| IBIS File LibisMaker.ibs
| Cadence Design Systems, Inc. 2024
[IBIS Ver]   7.0
[File name]   ln2-mh.ibs
[File rev]   1.7.1
[Date]   Wed Aug 12 20:25:11 PDT 2026
[Source]   Lattice Semiconductor Process
[Notes]   Device: LN2-MH-16
   CBG484   Final
   Device: LN2-MH-20
   CBG484   Final
   Lattice Semiconductor has worked hard to ensure the
   models below are accurate and complete.  However, the
   data below was generated using simulation of the
   input/output model files for the silicon.  Therefore,
   the data below is for reference and initial design
   purposes only.
   Lattice Semiconductor grants permission to use this
   data for use in printed circuit design using this
   Lattice programmable logic device.  Other use of this
   code, including the selling or duplication of any
   portion is strictly prohibited.
|   NAMING CONVENTION
   The IBIS [Model] header is limited by the specification to a
   total of characters.  With such a set of characters available
   for naming models it becomes important to attempt to
   meaningfully encode the IO standards so they fit within the
   twenty character limit.  It would seem that twenty characters
   would provide room enough for describing IO's.  However, the
   PLD IO structure continues to grow more and more complex.  The
   complexity is making the twenty characters insuffiently
   descriptive.  In order to overcome this issue the naming
   convention described below is implemented to resolve the issue.
The twenty character space is managed as follows:
   bbbvvvsdddprttmkoixx
   b = standard
   v = voltage (x.xx V)
   s = slew code
   d = drive (xx.x ma)
   p = pullmode code
   r = impedance
   t = termination code
   m = mipi hard dphy mode
   k = bank code
   o = diff resistor code
   i = diff  current code
   x = reserved
   standard
   lvcmos   lvc
   sstl135   ss1
   sstl135d   s1d
   hsul12   hs1
   hsul12d   h1d
   lvds   lvs
   lvdse   lve
   slvs   svs
   sublvds   slv
   sublvdse   sle
   mipi_dphy   mip
   pod   pod
   podd   pdd
   lvstl_i   ls1
   lvstl_ii   ls2
   lvstld_i   l1d
   lvstld_ii   l2d
   vref_driver   vr1
   slew
   na   a
   fast   f
   slow   s
   drive
   2   020
   4   040
   6   060
   8   080
   12   120
   50rs   r50
   34_ohm   034
   40_ohm   040
   48_ohm   048
   60_ohm   060
   80_ohm   080
   120_ohm   120
   240_ohm   240
   na   xxx
   pullmode
   none   a
   failsafe   a
   up   b
   down   c
   keeper   d
   i3c   i
   impedance
   off   a
   termination
   off   aa
   34   bb
   40   cc
   48   dd
   60   ee
   80   ff
   120   gg
   240   hh
   mipi hard dphy mode
   off   a
   lp   l
   hs   h
   bank
   wrio   a
   hpio   h
   differential resistor
   off   a
   100   b
   differential current
   NA   a
   2.0   b
   3.5   c
   Reserved   IO type
   in   input only
   ou   output
   io   I/O
   od   Open drain
   ic   Inverting differential input
   (signal name only)
   it   Non-Inverting differential
   input (signal name only)
   on   Inverting differential output
   (signal name only)
   op   Non-Inverting differential output
   (signal name only)
   bn   Inverting differential I/O
   (signal name only)
   bp   Non-Inverting differential I/O
   (signal name only)
   All the IO models are generated with pull mode set to none.
   Lattice Semiconductor Corporation
   5555 NE Moore Court
   Hillsboro, OR 97214
   U.S.A
   TEL: 1-800-Lattice (USA and Canada)
   408-826-6000 (other locations)
   All the IO models are generated with pull mode set to none.
   Lattice Semiconductor Corporation
   5555 NE Moore Court
   Hillsboro, OR 97214
   U.S.A
   TEL: 1-800-Lattice (USA and Canada)
   408-826-6000 (other locations)
   web: http://www.latticesemi.com/
   email: techsupport@latticesemi.com
[Disclaimer] This IBIS source code is intended as a design reference
   which illustrates how the Lattice Semiconductor device operates.
   It is the user's responsibility to verify their design for
   consistency and functionality through the use of formal
   verification methods.  Lattice Semiconductor provides no warranty
   regarding the use or functionality of this data.
[Copyright]  Copyright 2025 by Lattice Semiconductor Corporation
|   Component LN2-MH
[Component] LN2-MH
[Manufacturer] Lattice Semiconductor Corp.
[Package]
|CBG484_20ES1
| variable   typ   min   max
R_pkg   0.05332   0.013842   0.098293
L_pkg   2.82e-9   3.896e-10   5.244e-9
C_pkg   1.436e-12   6.976e-13   2.382e-12
|CBG484_16
| variable   typ   min   max
|R_pkg   0.3858   0.054089   0.93239
|L_pkg   2.783e-9   4.558e-10   6.119e-9
|C_pkg   1.392e-12   3.932e-13   2.869e-12
|CBG484_20
| variable   typ   min   max
|R_pkg   0.3858   0.054089   0.93239
|L_pkg   2.783e-9   4.558e-10   6.119e-9
|C_pkg   1.392e-12   3.932e-13   2.869e-12
[Pin]  signal_name   model_name   R_pin   L_pin   C_pin
1   lvc180axxxaaaaaaaain   lvc180axxxaaaaaaaain
2   lvc180axxxbaaaaaaain   lvc180axxxbaaaaaaain
3   lvc180axxxcaaaaaaain   lvc180axxxcaaaaaaain
4   lvc180axxxdaaaaaaain   lvc180axxxdaaaaaaain
5   lvc250axxxaaaaaaaain   lvc250axxxaaaaaaaain
6   lvc250axxxbaaaaaaain   lvc250axxxbaaaaaaain
7   lvc250axxxcaaaaaaain   lvc250axxxcaaaaaaain
8   lvc250axxxdaaaaaaain   lvc250axxxdaaaaaaain
9   lvc330axxxaaaaaaaain   lvc330axxxaaaaaaaain
10   lvc330axxxbaaaaaaain   lvc330axxxbaaaaaaain
11   lvc330axxxcaaaaaaain   lvc330axxxcaaaaaaain
12   lvc330axxxdaaaaaaain   lvc330axxxdaaaaaaain
13   lvc120axxxaaaaaaaain   lvc120axxxaaaaaaaain
14   lvc120axxxbaaaaaaain   lvc120axxxbaaaaaaain
15   lvc120axxxcaaaaaaain   lvc120axxxcaaaaaaain
16   lvc120axxxdaaaaaaain   lvc120axxxdaaaaaaain
17   lvc120axxxaaaaahaain   lvc120axxxaaaaahaain
18   lvc120axxxbaaaahaain   lvc120axxxbaaaahaain
19   lvc120axxxcaaaahaain   lvc120axxxcaaaahaain
20   lvc120axxxdaaaahaain   lvc120axxxdaaaahaain
21   lvc120axxxiaaaahaain   lvc120axxxiaaaahaain
22   lvc180axxxaaaaahaain   lvc180axxxaaaaahaain
23   lvc180axxxbaaaahaain   lvc180axxxbaaaahaain
24   lvc180axxxcaaaahaain   lvc180axxxcaaaahaain
25   lvc180axxxdaaaahaain   lvc180axxxdaaaahaain
26   lvc180axxxiaaaahaain   lvc180axxxiaaaahaain
27   lvc090axxxaaaaahaain   lvc090axxxaaaaahaain
28   lvc090axxxbaaaahaain   lvc090axxxbaaaahaain
29   lvc090axxxcaaaahaain   lvc090axxxcaaaahaain
30   lvc090axxxdaaaahaain   lvc090axxxdaaaahaain
31   lvc100axxxaaaaahaain   lvc100axxxaaaaahaain
32   lvc100axxxbaaaahaain   lvc100axxxbaaaahaain
33   lvc100axxxcaaaahaain   lvc100axxxcaaaahaain
34   lvc100axxxdaaaahaain   lvc100axxxdaaaahaain
35   ls1110axxxaabbahaain   ls1110axxxaabbahaain
36   ls1110axxxaaccahaain   ls1110axxxaaccahaain
37   ls1110axxxaaddahaain   ls1110axxxaaddahaain
38   ls1110axxxaaeeahaain   ls1110axxxaaeeahaain
39   ls1110axxxaaffahaain   ls1110axxxaaffahaain
40   ls1110axxxaaggahaain   ls1110axxxaaggahaain
41   ls1110axxxaahhahaain   ls1110axxxaahhahaain
42   ls2110axxxaabbahaain   ls2110axxxaabbahaain
43   ls2110axxxaaccahaain   ls2110axxxaaccahaain
44   ls2110axxxaaddahaain   ls2110axxxaaddahaain
45   ls2110axxxaaeeahaain   ls2110axxxaaeeahaain
46   ls2110axxxaaffahaain   ls2110axxxaaffahaain
47   ls2110axxxaaggahaain   ls2110axxxaaggahaain
48   ls2110axxxaahhahaain   ls2110axxxaahhahaain
49   hs1120axxxaaaaahaain   hs1120axxxaaaaahaain
50   hs1120axxxaaccahaain   hs1120axxxaaccahaain
51   hs1120axxxaaeeahaain   hs1120axxxaaeeahaain
52   pod110axxxaabbahaain   pod110axxxaabbahaain
53   pod110axxxaaccahaain   pod110axxxaaccahaain
54   pod110axxxaaddahaain   pod110axxxaaddahaain
55   pod110axxxaaeeahaain   pod110axxxaaeeahaain
56   pod110axxxaaffahaain   pod110axxxaaffahaain
57   pod110axxxaaggahaain   pod110axxxaaggahaain
58   pod110axxxaahhahaain   pod110axxxaahhahaain
59   pod120axxxaabbahaain   pod120axxxaabbahaain
60   pod120axxxaaccahaain   pod120axxxaaccahaain
61   pod120axxxaaddahaain   pod120axxxaaddahaain
62   pod120axxxaaeeahaain   pod120axxxaaeeahaain
63   pod120axxxaaffahaain   pod120axxxaaffahaain
64   pod120axxxaaggahaain   pod120axxxaaggahaain
65   pod120axxxaahhahaain   pod120axxxaahhahaain
66   ss1135axxxaaaaahaain   ss1135axxxaaaaahaain
67   ss1135axxxaaccahaain   ss1135axxxaaccahaain
68   ss1135axxxaaeeahaain   ss1135axxxaaeeahaain
69   l1d110axxxaabbahaait   l1d110axxxaabbahaain
70   l1d110axxxaabbahaaic   l1d110axxxaabbahaain
71   l1d110axxxaaccahaait   l1d110axxxaaccahaain
72   l1d110axxxaaccahaaic   l1d110axxxaaccahaain
73   l1d110axxxaaddahaait   l1d110axxxaaddahaain
74   l1d110axxxaaddahaaic   l1d110axxxaaddahaain
75   l1d110axxxaaeeahaait   l1d110axxxaaeeahaain
76   l1d110axxxaaeeahaaic   l1d110axxxaaeeahaain
77   l1d110axxxaaffahaait   l1d110axxxaaffahaain
78   l1d110axxxaaffahaaic   l1d110axxxaaffahaain
79   l1d110axxxaaggahaait   l1d110axxxaaggahaain
80   l1d110axxxaaggahaaic   l1d110axxxaaggahaain
81   l1d110axxxaahhahaait   l1d110axxxaahhahaain
82   l1d110axxxaahhahaaic   l1d110axxxaahhahaain
83   l2d110axxxaabbahaait   l2d110axxxaabbahaain
84   l2d110axxxaabbahaaic   l2d110axxxaabbahaain
85   l2d110axxxaaccahaait   l2d110axxxaaccahaain
86   l2d110axxxaaccahaaic   l2d110axxxaaccahaain
87   l2d110axxxaaddahaait   l2d110axxxaaddahaain
88   l2d110axxxaaddahaaic   l2d110axxxaaddahaain
89   l2d110axxxaaeeahaait   l2d110axxxaaeeahaain
90   l2d110axxxaaeeahaaic   l2d110axxxaaeeahaain
91   l2d110axxxaaffahaait   l2d110axxxaaffahaain
92   l2d110axxxaaffahaaic   l2d110axxxaaffahaain
93   l2d110axxxaaggahaait   l2d110axxxaaggahaain
94   l2d110axxxaaggahaaic   l2d110axxxaaggahaain
95   l2d110axxxaahhahaait   l2d110axxxaahhahaain
96   l2d110axxxaahhahaaic   l2d110axxxaahhahaain
97   h1d120axxxaaaaahaait   h1d120axxxaaaaahaain
98   h1d120axxxaaaaahaaic   h1d120axxxaaaaahaain
99   h1d120axxxaaaaahbait   h1d120axxxaaaaahbain
100   h1d120axxxaaaaahbaic   h1d120axxxaaaaahbain
101   h1d120axxxaaccahaait   h1d120axxxaaccahaain
102   h1d120axxxaaccahaaic   h1d120axxxaaccahaain
103   h1d120axxxaaccahbait   h1d120axxxaaccahbain
104   h1d120axxxaaccahbaic   h1d120axxxaaccahbain
105   h1d120axxxaaeeahaait   h1d120axxxaaeeahaain
106   h1d120axxxaaeeahaaic   h1d120axxxaaeeahaain
107   h1d120axxxaaeeahbait   h1d120axxxaaeeahbain
108   h1d120axxxaaeeahbaic   h1d120axxxaaeeahbain
109   pdd110axxxaabbahaait   pdd110axxxaabbahaain
110   pdd110axxxaabbahaaic   pdd110axxxaabbahaain
111   pdd110axxxaaccahaait   pdd110axxxaaccahaain
112   pdd110axxxaaccahaaic   pdd110axxxaaccahaain
113   pdd110axxxaaddahaait   pdd110axxxaaddahaain
114   pdd110axxxaaddahaaic   pdd110axxxaaddahaain
115   pdd110axxxaaeeahaait   pdd110axxxaaeeahaain
116   pdd110axxxaaeeahaaic   pdd110axxxaaeeahaain
117   pdd110axxxaaffahaait   pdd110axxxaaffahaain
118   pdd110axxxaaffahaaic   pdd110axxxaaffahaain
119   pdd110axxxaaggahaait   pdd110axxxaaggahaain
120   pdd110axxxaaggahaaic   pdd110axxxaaggahaain
121   pdd110axxxaahhahaait   pdd110axxxaahhahaain
122   pdd110axxxaahhahaaic   pdd110axxxaahhahaain
123   pdd120axxxaabbahaait   pdd120axxxaabbahaain
124   pdd120axxxaabbahaaic   pdd120axxxaabbahaain
125   pdd120axxxaaccahaait   pdd120axxxaaccahaain
126   pdd120axxxaaccahaaic   pdd120axxxaaccahaain
127   pdd120axxxaaddahaait   pdd120axxxaaddahaain
128   pdd120axxxaaddahaaic   pdd120axxxaaddahaain
129   pdd120axxxaaeeahaait   pdd120axxxaaeeahaain
130   pdd120axxxaaeeahaaic   pdd120axxxaaeeahaain
131   pdd120axxxaaffahaait   pdd120axxxaaffahaain
132   pdd120axxxaaffahaaic   pdd120axxxaaffahaain
133   pdd120axxxaaggahaait   pdd120axxxaaggahaain
134   pdd120axxxaaggahaaic   pdd120axxxaaggahaain
135   pdd120axxxaahhahaait   pdd120axxxaahhahaain
136   pdd120axxxaahhahaaic   pdd120axxxaahhahaain
137   s1d135axxxaaaaahaait   s1d135axxxaaaaahaain
138   s1d135axxxaaaaahaaic   s1d135axxxaaaaahaain
139   s1d135axxxaaaaahbait   s1d135axxxaaaaahbain
140   s1d135axxxaaaaahbaic   s1d135axxxaaaaahbain
141   s1d135axxxaaccahaait   s1d135axxxaaccahaain
142   s1d135axxxaaccahaaic   s1d135axxxaaccahaain
143   s1d135axxxaaccahbait   s1d135axxxaaccahbain
144   s1d135axxxaaccahbaic   s1d135axxxaaccahbain
145   s1d135axxxaaeeahaait   s1d135axxxaaeeahaain
146   s1d135axxxaaeeahaaic   s1d135axxxaaeeahaain
147   s1d135axxxaaeeahbait   s1d135axxxaaeeahbain
148   s1d135axxxaaeeahbaic   s1d135axxxaaeeahbain
149   slv180axxxaaaaahaait   slv180axxxaaaaahaain
150   slv180axxxaaaaahaaic   slv180axxxaaaaahaain
151   slv180axxxaaaaahbait   slv180axxxaaaaahbain
152   slv180axxxaaaaahbaic   slv180axxxaaaaahbain
153   svs120axxxaaaaahaait   svs120axxxaaaaahaain
154   svs120axxxaaaaahaaic   svs120axxxaaaaahaain
155   svs120axxxaaaaahbait   svs120axxxaaaaahbain
156   svs120axxxaaaaahbaic   svs120axxxaaaaahbain
157   mip120axxxaaaaahbait   mip120axxxaaaaahbain
158   mip120axxxaaaaahbaic   mip120axxxaaaaahbain
159   lvs180axxxaaaaahaait   lvs180axxxaaaaahaain
160   lvs180axxxaaaaahaaic   lvs180axxxaaaaahaain
161   lvs180axxxaaaaahbait   lvs180axxxaaaaahbain
162   lvs180axxxaaaaahbaic   lvs180axxxaaaaahbain
163   lvc120f040aaaaahaaou   lvc120f040aaaaahaaou
164   lvc120f080aaaaahaaou   lvc120f080aaaaahaaou
165   lvc120f120aaaaahaaou   lvc120f120aaaaahaaou
166   lvc120s040aaaaahaaou   lvc120s040aaaaahaaou
167   lvc120s080aaaaahaaou   lvc120s080aaaaahaaou
168   lvc120s120aaaaahaaou   lvc120s120aaaaahaaou
169   lvc180f040aaaaahaaou   lvc180f040aaaaahaaou
170   lvc180f080aaaaahaaou   lvc180f080aaaaahaaou
171   lvc180f120aaaaahaaou   lvc180f120aaaaahaaou
172   lvc180fr50aaaaahaaou   lvc180fr50aaaaahaaou
173   lvc180s040aaaaahaaou   lvc180s040aaaaahaaou
174   lvc180s080aaaaahaaou   lvc180s080aaaaahaaou
175   lvc180s120aaaaahaaou   lvc180s120aaaaahaaou
176   lvc180sr50aaaaahaaou   lvc180sr50aaaaahaaou
177   lvc090f020aaaaahaaou   lvc090f020aaaaahaaou
178   lvc090f040aaaaahaaou   lvc090f040aaaaahaaou
179   lvc090f080aaaaahaaou   lvc090f080aaaaahaaou
180   lvc090s020aaaaahaaou   lvc090s020aaaaahaaou
181   lvc090s040aaaaahaaou   lvc090s040aaaaahaaou
182   lvc090s080aaaaahaaou   lvc090s080aaaaahaaou
183   lvc100f020aaaaahaaou   lvc100f020aaaaahaaou
184   lvc100f040aaaaahaaou   lvc100f040aaaaahaaou
185   lvc100f080aaaaahaaou   lvc100f080aaaaahaaou
186   lvc100s020aaaaahaaou   lvc100s020aaaaahaaou
187   lvc100s040aaaaahaaou   lvc100s040aaaaahaaou
188   lvc100s080aaaaahaaou   lvc100s080aaaaahaaou
189   lvc180f040aaaaaaaaou   lvc180f040aaaaaaaaou
190   lvc180f080aaaaaaaaou   lvc180f080aaaaaaaaou
191   lvc180f120aaaaaaaaou   lvc180f120aaaaaaaaou
192   lvc180fr50aaaaaaaaou   lvc180fr50aaaaaaaaou
193   lvc180s040aaaaaaaaou   lvc180s040aaaaaaaaou
194   lvc180s080aaaaaaaaou   lvc180s080aaaaaaaaou
195   lvc180s120aaaaaaaaou   lvc180s120aaaaaaaaou
196   lvc180sr50aaaaaaaaou   lvc180sr50aaaaaaaaou
197   lvc250f040aaaaaaaaou   lvc250f040aaaaaaaaou
198   lvc250f080aaaaaaaaou   lvc250f080aaaaaaaaou
199   lvc250f120aaaaaaaaou   lvc250f120aaaaaaaaou
200   lvc250fr50aaaaaaaaou   lvc250fr50aaaaaaaaou
201   lvc250s040aaaaaaaaou   lvc250s040aaaaaaaaou
202   lvc250s080aaaaaaaaou   lvc250s080aaaaaaaaou
203   lvc250s120aaaaaaaaou   lvc250s120aaaaaaaaou
204   lvc250sr50aaaaaaaaou   lvc250sr50aaaaaaaaou
205   lvc330f040aaaaaaaaou   lvc330f040aaaaaaaaou
206   lvc330f080aaaaaaaaou   lvc330f080aaaaaaaaou
207   lvc330f120aaaaaaaaou   lvc330f120aaaaaaaaou
208   lvc330fr50aaaaaaaaou   lvc330fr50aaaaaaaaou
209   lvc330s040aaaaaaaaou   lvc330s040aaaaaaaaou
210   lvc330s080aaaaaaaaou   lvc330s080aaaaaaaaou
211   lvc330s120aaaaaaaaou   lvc330s120aaaaaaaaou
212   lvc330sr50aaaaaaaaou   lvc330sr50aaaaaaaaou
213   lvc120f060aaaaaaaaou   lvc120f060aaaaaaaaou
214   lvc120f080aaaaaaaaou   lvc120f080aaaaaaaaou
215   lvc120s060aaaaaaaaou   lvc120s060aaaaaaaaou
216   lvc120s080aaaaaaaaou   lvc120s080aaaaaaaaou
217   lve250f120aaaaaaaaop   lve250f120aaaaaaaaou
218   lve250f120aaaaaaaaon   lve250f120aaaaaaaaou
219   lve250s120aaaaaaaaop   lve250s120aaaaaaaaou
220   lve250s120aaaaaaaaon   lve250s120aaaaaaaaou
221   lvs180axxxaaaaahacop   lvs180axxxaaaaahacou
222   lvs180axxxaaaaahacon   lvs180axxxaaaaahacou
223   ls1110f034aaaaahaaou   ls1110f034aaaaahaaou
224   ls1110f040aaaaahaaou   ls1110f040aaaaahaaou
225   ls1110f048aaaaahaaou   ls1110f048aaaaahaaou
226   ls1110f060aaaaahaaou   ls1110f060aaaaahaaou
227   ls1110f080aaaaahaaou   ls1110f080aaaaahaaou
228   ls1110f120aaaaahaaou   ls1110f120aaaaahaaou
229   ls1110f240aaaaahaaou   ls1110f240aaaaahaaou
230   ls1110s034aaaaahaaou   ls1110s034aaaaahaaou
231   ls1110s040aaaaahaaou   ls1110s040aaaaahaaou
232   ls1110s048aaaaahaaou   ls1110s048aaaaahaaou
233   ls1110s060aaaaahaaou   ls1110s060aaaaahaaou
234   ls1110s080aaaaahaaou   ls1110s080aaaaahaaou
235   ls1110s120aaaaahaaou   ls1110s120aaaaahaaou
236   ls1110s240aaaaahaaou   ls1110s240aaaaahaaou
237   ls2110f034aaaaahaaou   ls2110f034aaaaahaaou
238   ls2110f040aaaaahaaou   ls2110f040aaaaahaaou
239   ls2110f048aaaaahaaou   ls2110f048aaaaahaaou
240   ls2110f060aaaaahaaou   ls2110f060aaaaahaaou
241   ls2110f080aaaaahaaou   ls2110f080aaaaahaaou
242   ls2110f120aaaaahaaou   ls2110f120aaaaahaaou
243   ls2110f240aaaaahaaou   ls2110f240aaaaahaaou
244   ls2110s034aaaaahaaou   ls2110s034aaaaahaaou
245   ls2110s040aaaaahaaou   ls2110s040aaaaahaaou
246   ls2110s048aaaaahaaou   ls2110s048aaaaahaaou
247   ls2110s060aaaaahaaou   ls2110s060aaaaahaaou
248   ls2110s080aaaaahaaou   ls2110s080aaaaahaaou
249   ls2110s120aaaaahaaou   ls2110s120aaaaahaaou
250   ls2110s240aaaaahaaou   ls2110s240aaaaahaaou
251   hs1120f034aaaaahaaou   hs1120f034aaaaahaaou
252   hs1120f040aaaaahaaou   hs1120f040aaaaahaaou
253   hs1120f048aaaaahaaou   hs1120f048aaaaahaaou
254   hs1120s034aaaaahaaou   hs1120s034aaaaahaaou
255   hs1120s040aaaaahaaou   hs1120s040aaaaahaaou
256   hs1120s048aaaaahaaou   hs1120s048aaaaahaaou
257   pod110f034aaaaahaaou   pod110f034aaaaahaaou
258   pod110f040aaaaahaaou   pod110f040aaaaahaaou
259   pod110f048aaaaahaaou   pod110f048aaaaahaaou
260   pod110f060aaaaahaaou   pod110f060aaaaahaaou
261   pod110f080aaaaahaaou   pod110f080aaaaahaaou
262   pod110f120aaaaahaaou   pod110f120aaaaahaaou
263   pod110f240aaaaahaaou   pod110f240aaaaahaaou
264   pod110s034aaaaahaaou   pod110s034aaaaahaaou
265   pod110s040aaaaahaaou   pod110s040aaaaahaaou
266   pod110s048aaaaahaaou   pod110s048aaaaahaaou
267   pod110s060aaaaahaaou   pod110s060aaaaahaaou
268   pod110s080aaaaahaaou   pod110s080aaaaahaaou
269   pod110s120aaaaahaaou   pod110s120aaaaahaaou
270   pod110s240aaaaahaaou   pod110s240aaaaahaaou
271   pod120f034aaaaahaaou   pod120f034aaaaahaaou
272   pod120f040aaaaahaaou   pod120f040aaaaahaaou
273   pod120f048aaaaahaaou   pod120f048aaaaahaaou
274   pod120f060aaaaahaaou   pod120f060aaaaahaaou
275   pod120f080aaaaahaaou   pod120f080aaaaahaaou
276   pod120f120aaaaahaaou   pod120f120aaaaahaaou
277   pod120f240aaaaahaaou   pod120f240aaaaahaaou
278   pod120s034aaaaahaaou   pod120s034aaaaahaaou
279   pod120s040aaaaahaaou   pod120s040aaaaahaaou
280   pod120s048aaaaahaaou   pod120s048aaaaahaaou
281   pod120s060aaaaahaaou   pod120s060aaaaahaaou
282   pod120s080aaaaahaaou   pod120s080aaaaahaaou
283   pod120s120aaaaahaaou   pod120s120aaaaahaaou
284   pod120s240aaaaahaaou   pod120s240aaaaahaaou
285   ss1135f034aaaaahaaou   ss1135f034aaaaahaaou
286   ss1135f040aaaaahaaou   ss1135f040aaaaahaaou
287   ss1135s034aaaaahaaou   ss1135s034aaaaahaaou
288   ss1135s040aaaaahaaou   ss1135s040aaaaahaaou
289   l1d110f034aaaaahaaop   l1d110f034aaaaahaaou
290   l1d110f034aaaaahaaon   l1d110f034aaaaahaaou
291   l1d110f040aaaaahaaop   l1d110f040aaaaahaaou
292   l1d110f040aaaaahaaon   l1d110f040aaaaahaaou
293   l1d110f048aaaaahaaop   l1d110f048aaaaahaaou
294   l1d110f048aaaaahaaon   l1d110f048aaaaahaaou
295   l1d110f060aaaaahaaop   l1d110f060aaaaahaaou
296   l1d110f060aaaaahaaon   l1d110f060aaaaahaaou
297   l1d110f080aaaaahaaop   l1d110f080aaaaahaaou
298   l1d110f080aaaaahaaon   l1d110f080aaaaahaaou
299   l1d110f120aaaaahaaop   l1d110f120aaaaahaaou
300   l1d110f120aaaaahaaon   l1d110f120aaaaahaaou
301   l1d110f240aaaaahaaop   l1d110f240aaaaahaaou
302   l1d110f240aaaaahaaon   l1d110f240aaaaahaaou
303   l1d110s034aaaaahaaop   l1d110s034aaaaahaaou
304   l1d110s034aaaaahaaon   l1d110s034aaaaahaaou
305   l1d110s040aaaaahaaop   l1d110s040aaaaahaaou
306   l1d110s040aaaaahaaon   l1d110s040aaaaahaaou
307   l1d110s048aaaaahaaop   l1d110s048aaaaahaaou
308   l1d110s048aaaaahaaon   l1d110s048aaaaahaaou
309   l1d110s060aaaaahaaop   l1d110s060aaaaahaaou
310   l1d110s060aaaaahaaon   l1d110s060aaaaahaaou
311   l1d110s080aaaaahaaop   l1d110s080aaaaahaaou
312   l1d110s080aaaaahaaon   l1d110s080aaaaahaaou
313   l1d110s120aaaaahaaop   l1d110s120aaaaahaaou
314   l1d110s120aaaaahaaon   l1d110s120aaaaahaaou
315   l1d110s240aaaaahaaop   l1d110s240aaaaahaaou
316   l1d110s240aaaaahaaon   l1d110s240aaaaahaaou
317   l2d110f034aaaaahaaop   l2d110f034aaaaahaaou
318   l2d110f034aaaaahaaon   l2d110f034aaaaahaaou
319   l2d110f040aaaaahaaop   l2d110f040aaaaahaaou
320   l2d110f040aaaaahaaon   l2d110f040aaaaahaaou
321   l2d110f048aaaaahaaop   l2d110f048aaaaahaaou
322   l2d110f048aaaaahaaon   l2d110f048aaaaahaaou
323   l2d110f060aaaaahaaop   l2d110f060aaaaahaaou
324   l2d110f060aaaaahaaon   l2d110f060aaaaahaaou
325   l2d110f080aaaaahaaop   l2d110f080aaaaahaaou
326   l2d110f080aaaaahaaon   l2d110f080aaaaahaaou
327   l2d110f120aaaaahaaop   l2d110f120aaaaahaaou
328   l2d110f120aaaaahaaon   l2d110f120aaaaahaaou
329   l2d110f240aaaaahaaop   l2d110f240aaaaahaaou
330   l2d110f240aaaaahaaon   l2d110f240aaaaahaaou
331   l2d110s034aaaaahaaop   l2d110s034aaaaahaaou
332   l2d110s034aaaaahaaon   l2d110s034aaaaahaaou
333   l2d110s040aaaaahaaop   l2d110s040aaaaahaaou
334   l2d110s040aaaaahaaon   l2d110s040aaaaahaaou
335   l2d110s048aaaaahaaop   l2d110s048aaaaahaaou
336   l2d110s048aaaaahaaon   l2d110s048aaaaahaaou
337   l2d110s060aaaaahaaop   l2d110s060aaaaahaaou
338   l2d110s060aaaaahaaon   l2d110s060aaaaahaaou
339   l2d110s080aaaaahaaop   l2d110s080aaaaahaaou
340   l2d110s080aaaaahaaon   l2d110s080aaaaahaaou
341   l2d110s120aaaaahaaop   l2d110s120aaaaahaaou
342   l2d110s120aaaaahaaon   l2d110s120aaaaahaaou
343   l2d110s240aaaaahaaop   l2d110s240aaaaahaaou
344   l2d110s240aaaaahaaon   l2d110s240aaaaahaaou
345   h1d120f034aaaaahaaop   h1d120f034aaaaahaaou
346   h1d120f034aaaaahaaon   h1d120f034aaaaahaaou
347   h1d120f040aaaaahaaop   h1d120f040aaaaahaaou
348   h1d120f040aaaaahaaon   h1d120f040aaaaahaaou
349   h1d120f048aaaaahaaop   h1d120f048aaaaahaaou
350   h1d120f048aaaaahaaon   h1d120f048aaaaahaaou
351   h1d120s034aaaaahaaop   h1d120s034aaaaahaaou
352   h1d120s034aaaaahaaon   h1d120s034aaaaahaaou
353   h1d120s040aaaaahaaop   h1d120s040aaaaahaaou
354   h1d120s040aaaaahaaon   h1d120s040aaaaahaaou
355   h1d120s048aaaaahaaop   h1d120s048aaaaahaaou
356   h1d120s048aaaaahaaon   h1d120s048aaaaahaaou
357   pdd110f034aaaaahaaop   pdd110f034aaaaahaaou
358   pdd110f034aaaaahaaon   pdd110f034aaaaahaaou
359   pdd110f040aaaaahaaop   pdd110f040aaaaahaaou
360   pdd110f040aaaaahaaon   pdd110f040aaaaahaaou
361   pdd110f048aaaaahaaop   pdd110f048aaaaahaaou
362   pdd110f048aaaaahaaon   pdd110f048aaaaahaaou
363   pdd110f060aaaaahaaop   pdd110f060aaaaahaaou
364   pdd110f060aaaaahaaon   pdd110f060aaaaahaaou
365   pdd110f080aaaaahaaop   pdd110f080aaaaahaaou
366   pdd110f080aaaaahaaon   pdd110f080aaaaahaaou
367   pdd110f120aaaaahaaop   pdd110f120aaaaahaaou
368   pdd110f120aaaaahaaon   pdd110f120aaaaahaaou
369   pdd110f240aaaaahaaop   pdd110f240aaaaahaaou
370   pdd110f240aaaaahaaon   pdd110f240aaaaahaaou
371   pdd110s034aaaaahaaop   pdd110s034aaaaahaaou
372   pdd110s034aaaaahaaon   pdd110s034aaaaahaaou
373   pdd110s040aaaaahaaop   pdd110s040aaaaahaaou
374   pdd110s040aaaaahaaon   pdd110s040aaaaahaaou
375   pdd110s048aaaaahaaop   pdd110s048aaaaahaaou
376   pdd110s048aaaaahaaon   pdd110s048aaaaahaaou
377   pdd110s060aaaaahaaop   pdd110s060aaaaahaaou
378   pdd110s060aaaaahaaon   pdd110s060aaaaahaaou
379   pdd110s080aaaaahaaop   pdd110s080aaaaahaaou
380   pdd110s080aaaaahaaon   pdd110s080aaaaahaaou
381   pdd110s120aaaaahaaop   pdd110s120aaaaahaaou
382   pdd110s120aaaaahaaon   pdd110s120aaaaahaaou
383   pdd110s240aaaaahaaop   pdd110s240aaaaahaaou
384   pdd110s240aaaaahaaon   pdd110s240aaaaahaaou
385   pdd120f034aaaaahaaop   pdd120f034aaaaahaaou
386   pdd120f034aaaaahaaon   pdd120f034aaaaahaaou
387   pdd120f040aaaaahaaop   pdd120f040aaaaahaaou
388   pdd120f040aaaaahaaon   pdd120f040aaaaahaaou
389   pdd120f048aaaaahaaop   pdd120f048aaaaahaaou
390   pdd120f048aaaaahaaon   pdd120f048aaaaahaaou
391   pdd120f060aaaaahaaop   pdd120f060aaaaahaaou
392   pdd120f060aaaaahaaon   pdd120f060aaaaahaaou
393   pdd120f080aaaaahaaop   pdd120f080aaaaahaaou
394   pdd120f080aaaaahaaon   pdd120f080aaaaahaaou
395   pdd120f120aaaaahaaop   pdd120f120aaaaahaaou
396   pdd120f120aaaaahaaon   pdd120f120aaaaahaaou
397   pdd120f240aaaaahaaop   pdd120f240aaaaahaaou
398   pdd120f240aaaaahaaon   pdd120f240aaaaahaaou
399   pdd120s034aaaaahaaop   pdd120s034aaaaahaaou
400   pdd120s034aaaaahaaon   pdd120s034aaaaahaaou
401   pdd120s040aaaaahaaop   pdd120s040aaaaahaaou
402   pdd120s040aaaaahaaon   pdd120s040aaaaahaaou
403   pdd120s048aaaaahaaop   pdd120s048aaaaahaaou
404   pdd120s048aaaaahaaon   pdd120s048aaaaahaaou
405   pdd120s060aaaaahaaop   pdd120s060aaaaahaaou
406   pdd120s060aaaaahaaon   pdd120s060aaaaahaaou
407   pdd120s080aaaaahaaop   pdd120s080aaaaahaaou
408   pdd120s080aaaaahaaon   pdd120s080aaaaahaaou
409   pdd120s120aaaaahaaop   pdd120s120aaaaahaaou
410   pdd120s120aaaaahaaon   pdd120s120aaaaahaaou
411   pdd120s240aaaaahaaop   pdd120s240aaaaahaaou
412   pdd120s240aaaaahaaon   pdd120s240aaaaahaaou
413   s1d135f034aaaaahaaop   s1d135f034aaaaahaaou
414   s1d135f034aaaaahaaon   s1d135f034aaaaahaaou
415   s1d135f040aaaaahaaop   s1d135f040aaaaahaaou
416   s1d135f040aaaaahaaon   s1d135f040aaaaahaaou
417   s1d135s034aaaaahaaop   s1d135s034aaaaahaaou
418   s1d135s034aaaaahaaon   s1d135s034aaaaahaaou
419   s1d135s040aaaaahaaop   s1d135s040aaaaahaaou
420   s1d135s040aaaaahaaon   s1d135s040aaaaahaaou
421   sle180fr50aaaaaaaaop   sle180fr50aaaaaaaaou
422   sle180fr50aaaaaaaaon   sle180fr50aaaaaaaaou
423   sle180sr50aaaaaaaaop   sle180sr50aaaaaaaaou
424   sle180sr50aaaaaaaaon   sle180sr50aaaaaaaaou
425   sle180fr50aaaaahaaop   sle180fr50aaaaahaaou
426   sle180fr50aaaaahaaon   sle180fr50aaaaahaaou
427   sle180sr50aaaaahaaop   sle180sr50aaaaahaaou
428   sle180sr50aaaaahaaon   sle180sr50aaaaahaaou
429   svs120axxxaaaaahabop   svs120axxxaaaaahabou
430   svs120axxxaaaaahabon   svs120axxxaaaaahabou
431   lvc090f020aaaaahaaio   lvc090f020aaaaahaaio
432   lvc090f020baaaahaaio   lvc090f020baaaahaaio
433   lvc090f020caaaahaaio   lvc090f020caaaahaaio
434   lvc090f020daaaahaaio   lvc090f020daaaahaaio
435   lvc090f040aaaaahaaio   lvc090f040aaaaahaaio
436   lvc090f040baaaahaaio   lvc090f040baaaahaaio
437   lvc090f040caaaahaaio   lvc090f040caaaahaaio
438   lvc090f040daaaahaaio   lvc090f040daaaahaaio
439   lvc090f080aaaaahaaio   lvc090f080aaaaahaaio
440   lvc090f080baaaahaaio   lvc090f080baaaahaaio
441   lvc090f080caaaahaaio   lvc090f080caaaahaaio
442   lvc090f080daaaahaaio   lvc090f080daaaahaaio
443   lvc090s020aaaaahaaio   lvc090s020aaaaahaaio
444   lvc090s020baaaahaaio   lvc090s020baaaahaaio
445   lvc090s020caaaahaaio   lvc090s020caaaahaaio
446   lvc090s020daaaahaaio   lvc090s020daaaahaaio
447   lvc090s040aaaaahaaio   lvc090s040aaaaahaaio
448   lvc090s040baaaahaaio   lvc090s040baaaahaaio
449   lvc090s040caaaahaaio   lvc090s040caaaahaaio
450   lvc090s040daaaahaaio   lvc090s040daaaahaaio
451   lvc090s080aaaaahaaio   lvc090s080aaaaahaaio
452   lvc090s080baaaahaaio   lvc090s080baaaahaaio
453   lvc090s080caaaahaaio   lvc090s080caaaahaaio
454   lvc090s080daaaahaaio   lvc090s080daaaahaaio
455   lvc100f020aaaaahaaio   lvc100f020aaaaahaaio
456   lvc100f020baaaahaaio   lvc100f020baaaahaaio
457   lvc100f020caaaahaaio   lvc100f020caaaahaaio
458   lvc100f020daaaahaaio   lvc100f020daaaahaaio
459   lvc100f040aaaaahaaio   lvc100f040aaaaahaaio
460   lvc100f040baaaahaaio   lvc100f040baaaahaaio
461   lvc100f040caaaahaaio   lvc100f040caaaahaaio
462   lvc100f040daaaahaaio   lvc100f040daaaahaaio
463   lvc100f080aaaaahaaio   lvc100f080aaaaahaaio
464   lvc100f080baaaahaaio   lvc100f080baaaahaaio
465   lvc100f080caaaahaaio   lvc100f080caaaahaaio
466   lvc100f080daaaahaaio   lvc100f080daaaahaaio
467   lvc100s020aaaaahaaio   lvc100s020aaaaahaaio
468   lvc100s020baaaahaaio   lvc100s020baaaahaaio
469   lvc100s020caaaahaaio   lvc100s020caaaahaaio
470   lvc100s020daaaahaaio   lvc100s020daaaahaaio
471   lvc100s040aaaaahaaio   lvc100s040aaaaahaaio
472   lvc100s040baaaahaaio   lvc100s040baaaahaaio
473   lvc100s040caaaahaaio   lvc100s040caaaahaaio
474   lvc100s040daaaahaaio   lvc100s040daaaahaaio
475   lvc100s080aaaaahaaio   lvc100s080aaaaahaaio
476   lvc100s080baaaahaaio   lvc100s080baaaahaaio
477   lvc100s080caaaahaaio   lvc100s080caaaahaaio
478   lvc100s080daaaahaaio   lvc100s080daaaahaaio
479   lvc120f040aaaaahaaio   lvc120f040aaaaahaaio
480   lvc120f040baaaahaaio   lvc120f040baaaahaaio
481   lvc120f040caaaahaaio   lvc120f040caaaahaaio
482   lvc120f040daaaahaaio   lvc120f040daaaahaaio
483   lvc120f040iaaaahaaio   lvc120f040iaaaahaaio
484   lvc120f080aaaaahaaio   lvc120f080aaaaahaaio
485   lvc120f080baaaahaaio   lvc120f080baaaahaaio
486   lvc120f080caaaahaaio   lvc120f080caaaahaaio
487   lvc120f080daaaahaaio   lvc120f080daaaahaaio
488   lvc120f080iaaaahaaio   lvc120f080iaaaahaaio
489   lvc120f120aaaaahaaio   lvc120f120aaaaahaaio
490   lvc120f120baaaahaaio   lvc120f120baaaahaaio
491   lvc120f120caaaahaaio   lvc120f120caaaahaaio
492   lvc120f120daaaahaaio   lvc120f120daaaahaaio
493   lvc120f120iaaaahaaio   lvc120f120iaaaahaaio
494   lvc120s040aaaaahaaio   lvc120s040aaaaahaaio
495   lvc120s040baaaahaaio   lvc120s040baaaahaaio
496   lvc120s040caaaahaaio   lvc120s040caaaahaaio
497   lvc120s040daaaahaaio   lvc120s040daaaahaaio
498   lvc120s040iaaaahaaio   lvc120s040iaaaahaaio
499   lvc120s080aaaaahaaio   lvc120s080aaaaahaaio
500   lvc120s080baaaahaaio   lvc120s080baaaahaaio
501   lvc120s080caaaahaaio   lvc120s080caaaahaaio
502   lvc120s080daaaahaaio   lvc120s080daaaahaaio
503   lvc120s080iaaaahaaio   lvc120s080iaaaahaaio
504   lvc120s120aaaaahaaio   lvc120s120aaaaahaaio
505   lvc120s120baaaahaaio   lvc120s120baaaahaaio
506   lvc120s120caaaahaaio   lvc120s120caaaahaaio
507   lvc120s120daaaahaaio   lvc120s120daaaahaaio
508   lvc120s120iaaaahaaio   lvc120s120iaaaahaaio
509   lvc180f040aaaaahaaio   lvc180f040aaaaahaaio
510   lvc180f040baaaahaaio   lvc180f040baaaahaaio
511   lvc180f040caaaahaaio   lvc180f040caaaahaaio
512   lvc180f040daaaahaaio   lvc180f040daaaahaaio
513   lvc180f040iaaaahaaio   lvc180f040iaaaahaaio
514   lvc180f080aaaaahaaio   lvc180f080aaaaahaaio
515   lvc180f080baaaahaaio   lvc180f080baaaahaaio
516   lvc180f080caaaahaaio   lvc180f080caaaahaaio
517   lvc180f080daaaahaaio   lvc180f080daaaahaaio
518   lvc180f080iaaaahaaio   lvc180f080iaaaahaaio
519   lvc180f120aaaaahaaio   lvc180f120aaaaahaaio
520   lvc180f120baaaahaaio   lvc180f120baaaahaaio
521   lvc180f120caaaahaaio   lvc180f120caaaahaaio
522   lvc180f120daaaahaaio   lvc180f120daaaahaaio
523   lvc180f120iaaaahaaio   lvc180f120iaaaahaaio
524   lvc180fr50aaaaahaaio   lvc180fr50aaaaahaaio
525   lvc180fr50baaaahaaio   lvc180fr50baaaahaaio
526   lvc180fr50caaaahaaio   lvc180fr50caaaahaaio
527   lvc180fr50daaaahaaio   lvc180fr50daaaahaaio
528   lvc180fr50iaaaahaaio   lvc180fr50iaaaahaaio
529   lvc180s040aaaaahaaio   lvc180s040aaaaahaaio
530   lvc180s040baaaahaaio   lvc180s040baaaahaaio
531   lvc180s040caaaahaaio   lvc180s040caaaahaaio
532   lvc180s040daaaahaaio   lvc180s040daaaahaaio
533   lvc180s040iaaaahaaio   lvc180s040iaaaahaaio
534   lvc180s080aaaaahaaio   lvc180s080aaaaahaaio
535   lvc180s080baaaahaaio   lvc180s080baaaahaaio
536   lvc180s080caaaahaaio   lvc180s080caaaahaaio
537   lvc180s080daaaahaaio   lvc180s080daaaahaaio
538   lvc180s080iaaaahaaio   lvc180s080iaaaahaaio
539   lvc180s120aaaaahaaio   lvc180s120aaaaahaaio
540   lvc180s120baaaahaaio   lvc180s120baaaahaaio
541   lvc180s120caaaahaaio   lvc180s120caaaahaaio
542   lvc180s120daaaahaaio   lvc180s120daaaahaaio
543   lvc180s120iaaaahaaio   lvc180s120iaaaahaaio
544   lvc180sr50aaaaahaaio   lvc180sr50aaaaahaaio
545   lvc180sr50baaaahaaio   lvc180sr50baaaahaaio
546   lvc180sr50caaaahaaio   lvc180sr50caaaahaaio
547   lvc180sr50daaaahaaio   lvc180sr50daaaahaaio
548   lvc180sr50iaaaahaaio   lvc180sr50iaaaahaaio
549   ss1135f040aaaaahaaio   ss1135f040aaaaahaaio
550   ss1135s040aaaaahaaio   ss1135s040aaaaahaaio
551   ss1135f040aaccahaaio   ss1135f040aaccahaaio
552   ss1135s034aaaaahaaio   ss1135s034aaaaahaaio
553   ss1135f040aaeeahaaio   ss1135f040aaeeahaaio
554   ss1135s040aaccahaaio   ss1135s040aaccahaaio
555   ss1135s034aaccahaaio   ss1135s034aaccahaaio
556   ss1135s034aaeeahaaio   ss1135s034aaeeahaaio
557   ss1135f034aaeeahaaio   ss1135f034aaeeahaaio
558   ss1135f034aaccahaaio   ss1135f034aaccahaaio
559   ss1135f034aaaaahaaio   ss1135f034aaaaahaaio
560   ss1135s040aaeeahaaio   ss1135s040aaeeahaaio
561   s1d135s040aaeeahaabp   s1d135s040aaeeahaaio
562   s1d135s040aaeeahaabn   s1d135s040aaeeahaaio
563   s1d135s034aaaaahaabp   s1d135s034aaaaahaaio
564   s1d135s034aaaaahaabn   s1d135s034aaaaahaaio
565   s1d135f034aaaaahaabp   s1d135f034aaaaahaaio
566   s1d135f034aaaaahaabn   s1d135f034aaaaahaaio
567   s1d135s034aaccahaabp   s1d135s034aaccahaaio
568   s1d135s034aaccahaabn   s1d135s034aaccahaaio
569   s1d135s034aaeeahaabp   s1d135s034aaeeahaaio
570   s1d135s034aaeeahaabn   s1d135s034aaeeahaaio
571   s1d135f034aaccahaabp   s1d135f034aaccahaaio
572   s1d135f034aaccahaabn   s1d135f034aaccahaaio
573   s1d135s040aaccahaabp   s1d135s040aaccahaaio
574   s1d135s040aaccahaabn   s1d135s040aaccahaaio
575   s1d135f040aaeeahaabp   s1d135f040aaeeahaaio
576   s1d135f040aaeeahaabn   s1d135f040aaeeahaaio
577   s1d135f034aaeeahaabp   s1d135f034aaeeahaaio
578   s1d135f034aaeeahaabn   s1d135f034aaeeahaaio
579   s1d135f040aaaaahaabp   s1d135f040aaaaahaaio
580   s1d135f040aaaaahaabn   s1d135f040aaaaahaaio
581   s1d135f040aaccahaabp   s1d135f040aaccahaaio
582   s1d135f040aaccahaabn   s1d135f040aaccahaaio
583   s1d135s040aaaaahaabp   s1d135s040aaaaahaaio
584   s1d135s040aaaaahaabn   s1d135s040aaaaahaaio
585   mip120a020aaaahhbbbp   mip120a020aaaahhbbio
586   mip120a020aaaahhbbbn   mip120a020aaaahhbbio
587   mip120a020aaaalhabio   mip120a020aaaalhabio
588   lvs180axxxaaaaahbcbp   lvs180axxxaaaaahbcio
589   lvs180axxxaaaaahbcbn   lvs180axxxaaaaahbcio
590   hs1120f034aaaaahaaio   hs1120f034aaaaahaaio
591   hs1120f048aaeeahaaio   hs1120f048aaeeahaaio
592   hs1120s034aaccahaaio   hs1120s034aaccahaaio
593   hs1120s034aaeeahaaio   hs1120s034aaeeahaaio
594   hs1120s040aaaaahaaio   hs1120s040aaaaahaaio
595   hs1120s048aaccahaaio   hs1120s048aaccahaaio
596   hs1120s034aaaaahaaio   hs1120s034aaaaahaaio
597   hs1120f040aaccahaaio   hs1120f040aaccahaaio
598   hs1120f048aaaaahaaio   hs1120f048aaaaahaaio
599   hs1120s048aaeeahaaio   hs1120s048aaeeahaaio
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[Diff pin]  inv_pin  vdiff  tdelay_typ  tdelay_min  tdelay_max
69   70   0.1   0.0s   0.0s   0.0s
71   72   0.1   0.0s   0.0s   0.0s
73   74   0.1   0.0s   0.0s   0.0s
75   76   0.1   0.0s   0.0s   0.0s
77   78   0.1   0.0s   0.0s   0.0s
79   80   0.1   0.0s   0.0s   0.0s
81   82   0.1   0.0s   0.0s   0.0s
83   84   0.1   0.0s   0.0s   0.0s
85   86   0.1   0.0s   0.0s   0.0s
87   88   0.1   0.0s   0.0s   0.0s
89   90   0.1   0.0s   0.0s   0.0s
91   92   0.1   0.0s   0.0s   0.0s
93   94   0.1   0.0s   0.0s   0.0s
95   96   0.1   0.0s   0.0s   0.0s
97   98   0.1   0.0s   0.0s   0.0s
99   100   0.1   0.0s   0.0s   0.0s
101   102   0.1   0.0s   0.0s   0.0s
103   104   0.1   0.0s   0.0s   0.0s
105   106   0.1   0.0s   0.0s   0.0s
107   108   0.1   0.0s   0.0s   0.0s
109   110   NA   NA   NA   NA
111   112   NA   NA   NA   NA
113   114   NA   NA   NA   NA
115   116   NA   NA   NA   NA
117   118   NA   NA   NA   NA
119   120   NA   NA   NA   NA
121   122   NA   NA   NA   NA
123   124   NA   NA   NA   NA
125   126   NA   NA   NA   NA
127   128   NA   NA   NA   NA
129   130   NA   NA   NA   NA
131   132   NA   NA   NA   NA
133   134   NA   NA   NA   NA
135   136   NA   NA   NA   NA
137   138   0.1   0.0s   0.0s   0.0s
139   140   0.1   0.0s   0.0s   0.0s
141   142   0.1   0.0s   0.0s   0.0s
143   144   0.1   0.0s   0.0s   0.0s
145   146   0.1   0.0s   0.0s   0.0s
147   148   0.1   0.0s   0.0s   0.0s
149   150   0.09   0.0s   0.0s   0.0s
151   152   0.09   0.0s   0.0s   0.0s
153   154   0.07   0.0s   0.0s   0.0s
155   156   0.07   0.0s   0.0s   0.0s
157   158   NA   NA   NA   NA
159   160   0.1   0.0s   0.0s   0.0s
161   162   0.1   0.0s   0.0s   0.0s
217   218   NA   NA   NA   NA
219   220   NA   NA   NA   NA
221   222   NA   NA   NA   NA
289   290   NA   NA   NA   NA
291   292   NA   NA   NA   NA
293   294   NA   NA   NA   NA
295   296   NA   NA   NA   NA
297   298   NA   NA   NA   NA
299   300   NA   NA   NA   NA
301   302   NA   NA   NA   NA
303   304   NA   NA   NA   NA
305   306   NA   NA   NA   NA
307   308   NA   NA   NA   NA
309   310   NA   NA   NA   NA
311   312   NA   NA   NA   NA
313   314   NA   NA   NA   NA
315   316   NA   NA   NA   NA
317   318   NA   NA   NA   NA
319   320   NA   NA   NA   NA
321   322   NA   NA   NA   NA
323   324   NA   NA   NA   NA
325   326   NA   NA   NA   NA
327   328   NA   NA   NA   NA
329   330   NA   NA   NA   NA
331   332   NA   NA   NA   NA
333   334   NA   NA   NA   NA
335   336   NA   NA   NA   NA
337   338   NA   NA   NA   NA
339   340   NA   NA   NA   NA
341   342   NA   NA   NA   NA
343   344   NA   NA   NA   NA
345   346   NA   NA   NA   NA
347   348   NA   NA   NA   NA
349   350   NA   NA   NA   NA
351   352   NA   NA   NA   NA
353   354   NA   NA   NA   NA
355   356   NA   NA   NA   NA
357   358   NA   NA   NA   NA
359   360   NA   NA   NA   NA
361   362   NA   NA   NA   NA
363   364   NA   NA   NA   NA
365   366   NA   NA   NA   NA
367   368   NA   NA   NA   NA
369   370   NA   NA   NA   NA
371   372   NA   NA   NA   NA
373   374   NA   NA   NA   NA
375   376   NA   NA   NA   NA
377   378   NA   NA   NA   NA
379   380   NA   NA   NA   NA
381   382   NA   NA   NA   NA
383   384   NA   NA   NA   NA
385   386   NA   NA   NA   NA
387   388   NA   NA   NA   NA
389   390   NA   NA   NA   NA
391   392   NA   NA   NA   NA
393   394   NA   NA   NA   NA
395   396   NA   NA   NA   NA
397   398   NA   NA   NA   NA
399   400   NA   NA   NA   NA
401   402   NA   NA   NA   NA
403   404   NA   NA   NA   NA
405   406   NA   NA   NA   NA
407   408   NA   NA   NA   NA
409   410   NA   NA   NA   NA
411   412   NA   NA   NA   NA
413   414   NA   NA   NA   NA
415   416   NA   NA   NA   NA
417   418   NA   NA   NA   NA
419   420   NA   NA   NA   NA
421   422   NA   NA   NA   NA
423   424   NA   NA   NA   NA
425   426   NA   NA   NA   NA
427   428   NA   NA   NA   NA
429   430   NA   NA   NA   NA
561   562   NA   NA   NA   NA
563   564   NA   NA   NA   NA
565   566   NA   NA   NA   NA
567   568   NA   NA   NA   NA
569   570   NA   NA   NA   NA
571   572   NA   NA   NA   NA
573   574   NA   NA   NA   NA
575   576   NA   NA   NA   NA
577   578   NA   NA   NA   NA
579   580   NA   NA   NA   NA
581   582   NA   NA   NA   NA
583   584   NA   NA   NA   NA
585   586   NA   NA   NA   NA
588   589   NA   NA   NA   NA
608   609   NA   NA   NA   NA
610   611   NA   NA   NA   NA
612   613   NA   NA   NA   NA
614   615   NA   NA   NA   NA
616   617   NA   NA   NA   NA
618   619   NA   NA   NA   NA
620   621   NA   NA   NA   NA
622   623   NA   NA   NA   NA
624   625   NA   NA   NA   NA
626   627   NA   NA   NA   NA
628   629   NA   NA   NA   NA
630   631   NA   NA   NA   NA
632   633   NA   NA   NA   NA
634   635   NA   NA   NA   NA
636   637   NA   NA   NA   NA
638   639   NA   NA   NA   NA
640   641   NA   NA   NA   NA
642   643   NA   NA   NA   NA
644   645   NA   NA   NA   NA
646   647   NA   NA   NA   NA
648   649   NA   NA   NA   NA
650   651   NA   NA   NA   NA
652   653   NA   NA   NA   NA
654   655   NA   NA   NA   NA
656   657   NA   NA   NA   NA
658   659   NA   NA   NA   NA
660   661   NA   NA   NA   NA
662   663   NA   NA   NA   NA
664   665   NA   NA   NA   NA
666   667   NA   NA   NA   NA
668   669   NA   NA   NA   NA
670   671   NA   NA   NA   NA
672   673   NA   NA   NA   NA
674   675   NA   NA   NA   NA
676   677   NA   NA   NA   NA
678   679   NA   NA   NA   NA
778   779   NA   NA   NA   NA
780   781   NA   NA   NA   NA
782   783   NA   NA   NA   NA
784   785   NA   NA   NA   NA
786   787   NA   NA   NA   NA
788   789   NA   NA   NA   NA
790   791   NA   NA   NA   NA
792   793   NA   NA   NA   NA
794   795   NA   NA   NA   NA
796   797   NA   NA   NA   NA
798   799   NA   NA   NA   NA
800   801   NA   NA   NA   NA
802   803   NA   NA   NA   NA
804   805   NA   NA   NA   NA
806   807   NA   NA   NA   NA
808   809   NA   NA   NA   NA
810   811   NA   NA   NA   NA
812   813   NA   NA   NA   NA
814   815   NA   NA   NA   NA
816   817   NA   NA   NA   NA
818   819   NA   NA   NA   NA
820   821   NA   NA   NA   NA
822   823   NA   NA   NA   NA
824   825   NA   NA   NA   NA
826   827   NA   NA   NA   NA
828   829   NA   NA   NA   NA
830   831   NA   NA   NA   NA
832   833   NA   NA   NA   NA
834   835   NA   NA   NA   NA
836   837   NA   NA   NA   NA
838   839   NA   NA   NA   NA
840   841   NA   NA   NA   NA
842   843   NA   NA   NA   NA
844   845   NA   NA   NA   NA
846   847   NA   NA   NA   NA
848   849   NA   NA   NA   NA
850   851   NA   NA   NA   NA
852   853   NA   NA   NA   NA
854   855   NA   NA   NA   NA
856   857   NA   NA   NA   NA
858   859   NA   NA   NA   NA
860   861   NA   NA   NA   NA
862   863   NA   NA   NA   NA
864   865   NA   NA   NA   NA
866   867   NA   NA   NA   NA
868   869   NA   NA   NA   NA
870   871   NA   NA   NA   NA
872   873   NA   NA   NA   NA
874   875   NA   NA   NA   NA
876   877   NA   NA   NA   NA
878   879   NA   NA   NA   NA
880   881   NA   NA   NA   NA
882   883   NA   NA   NA   NA
884   885   NA   NA   NA   NA
886   887   NA   NA   NA   NA
888   889   NA   NA   NA   NA
890   891   NA   NA   NA   NA
892   893   NA   NA   NA   NA
894   895   NA   NA   NA   NA
896   897   NA   NA   NA   NA
898   899   NA   NA   NA   NA
900   901   NA   NA   NA   NA
902   903   NA   NA   NA   NA
904   905   NA   NA   NA   NA
906   907   NA   NA   NA   NA
908   909   NA   NA   NA   NA
910   911   NA   NA   NA   NA
912   913   NA   NA   NA   NA
914   915   NA   NA   NA   NA
916   917   NA   NA   NA   NA
918   919   NA   NA   NA   NA
920   921   NA   NA   NA   NA
922   923   NA   NA   NA   NA
924   925   NA   NA   NA   NA
926   927   NA   NA   NA   NA
928   929   NA   NA   NA   NA
930   931   NA   NA   NA   NA
932   933   NA   NA   NA   NA
934   935   NA   NA   NA   NA
936   937   NA   NA   NA   NA
938   939   NA   NA   NA   NA
940   941   NA   NA   NA   NA
942   943   NA   NA   NA   NA
944   945   NA   NA   NA   NA
946   947   NA   NA   NA   NA
948   949   NA   NA   NA   NA
950   951   NA   NA   NA   NA
952   953   NA   NA   NA   NA
954   955   NA   NA   NA   NA
956   957   NA   NA   NA   NA
958   959   NA   NA   NA   NA
960   961   NA   NA   NA   NA
962   963   NA   NA   NA   NA
964   965   NA   NA   NA   NA
966   967   NA   NA   NA   NA
968   969   NA   NA   NA   NA
970   971   NA   NA   NA   NA
972   973   NA   NA   NA   NA
1072   1073   NA   NA   NA   NA
1074   1075   NA   NA   NA   NA
1076   1077   NA   NA   NA   NA
1078   1079   NA   NA   NA   NA
1080   1081   NA   NA   NA   NA
1082   1083   NA   NA   NA   NA
1084   1085   NA   NA   NA   NA
1086   1087   NA   NA   NA   NA
1088   1089   NA   NA   NA   NA
1090   1091   NA   NA   NA   NA
1092   1093   NA   NA   NA   NA
1094   1095   NA   NA   NA   NA
1096   1097   NA   NA   NA   NA
1098   1099   NA   NA   NA   NA
1100   1101   NA   NA   NA   NA
1102   1103   NA   NA   NA   NA
1104   1105   NA   NA   NA   NA
1106   1107   NA   NA   NA   NA
1108   1109   NA   NA   NA   NA
1110   1111   NA   NA   NA   NA
1112   1113   NA   NA   NA   NA
1114   1115   NA   NA   NA   NA
1116   1117   NA   NA   NA   NA
1118   1119   NA   NA   NA   NA
1120   1121   NA   NA   NA   NA
1122   1123   NA   NA   NA   NA
1124   1125   NA   NA   NA   NA
1126   1127   NA   NA   NA   NA
1128   1129   NA   NA   NA   NA
1130   1131   NA   NA   NA   NA
1132   1133   NA   NA   NA   NA
1134   1135   NA   NA   NA   NA
1136   1137   NA   NA   NA   NA
1138   1139   NA   NA   NA   NA
1140   1141   NA   NA   NA   NA
1142   1143   NA   NA   NA   NA
1144   1145   NA   NA   NA   NA
1146   1147   NA   NA   NA   NA
1148   1149   NA   NA   NA   NA
1150   1151   NA   NA   NA   NA
1152   1153   NA   NA   NA   NA
1154   1155   NA   NA   NA   NA
1156   1157   NA   NA   NA   NA
1158   1159   NA   NA   NA   NA
1160   1161   NA   NA   NA   NA
1162   1163   NA   NA   NA   NA
1164   1165   NA   NA   NA   NA
1166   1167   NA   NA   NA   NA
1168   1169   NA   NA   NA   NA
1170   1171   NA   NA   NA   NA
1172   1173   NA   NA   NA   NA
1174   1175   NA   NA   NA   NA
1176   1177   NA   NA   NA   NA
1178   1179   NA   NA   NA   NA
1180   1181   NA   NA   NA   NA
1182   1183   NA   NA   NA   NA
1184   1185   NA   NA   NA   NA
1186   1187   NA   NA   NA   NA
1188   1189   NA   NA   NA   NA
1190   1191   NA   NA   NA   NA
1192   1193   NA   NA   NA   NA
1194   1195   NA   NA   NA   NA
1196   1197   NA   NA   NA   NA
1198   1199   NA   NA   NA   NA
1200   1201   NA   NA   NA   NA
1202   1203   NA   NA   NA   NA
1204   1205   NA   NA   NA   NA
1206   1207   NA   NA   NA   NA
1208   1209   NA   NA   NA   NA
1210   1211   NA   NA   NA   NA
1212   1213   NA   NA   NA   NA
1214   1215   NA   NA   NA   NA
1216   1217   NA   NA   NA   NA
1218   1219   NA   NA   NA   NA
1220   1221   NA   NA   NA   NA
1222   1223   NA   NA   NA   NA
1224   1225   NA   NA   NA   NA
1226   1227   NA   NA   NA   NA
1228   1229   NA   NA   NA   NA
1230   1231   NA   NA   NA   NA
1232   1233   NA   NA   NA   NA
1234   1235   NA   NA   NA   NA
1236   1237   NA   NA   NA   NA
1238   1239   NA   NA   NA   NA
1240   1241   NA   NA   NA   NA
1242   1243   NA   NA   NA   NA
1244   1245   NA   NA   NA   NA
1246   1247   NA   NA   NA   NA
1248   1249   NA   NA   NA   NA
1250   1251   NA   NA   NA   NA
1252   1253   NA   NA   NA   NA
1254   1255   NA   NA   NA   NA
1256   1257   NA   NA   NA   NA
1258   1259   NA   NA   NA   NA
1260   1261   NA   NA   NA   NA
1262   1263   NA   NA   NA   NA
1264   1265   NA   NA   NA   NA
1266   1267   NA   NA   NA   NA
1268   1269   NA   NA   NA   NA
1270   1271   NA   NA   NA   NA
1272   1273   NA   NA   NA   NA
1274   1275   NA   NA   NA   NA
1276   1277   NA   NA   NA   NA
1278   1279   NA   NA   NA   NA
1280   1281   NA   NA   NA   NA
1282   1283   NA   NA   NA   NA
1284   1285   NA   NA   NA   NA
1286   1287   NA   NA   NA   NA
1288   1289   NA   NA   NA   NA
1290   1291   NA   NA   NA   NA
1292   1293   NA   NA   NA   NA
1294   1295   NA   NA   NA   NA
1296   1297   NA   NA   NA   NA
1298   1299   NA   NA   NA   NA
1300   1301   NA   NA   NA   NA
1302   1303   NA   NA   NA   NA
1304   1305   NA   NA   NA   NA
1306   1307   NA   NA   NA   NA
1308   1309   NA   NA   NA   NA
1310   1311   NA   NA   NA   NA
1312   1313   NA   NA   NA   NA
1314   1315   NA   NA   NA   NA
1316   1317   NA   NA   NA   NA
1318   1319   NA   NA   NA   NA
1320   1321   NA   NA   NA   NA
1322   1323   NA   NA   NA   NA
1324   1325   NA   NA   NA   NA
1326   1327   NA   NA   NA   NA
1328   1329   NA   NA   NA   NA
1330   1331   NA   NA   NA   NA
1332   1333   NA   NA   NA   NA
1334   1335   NA   NA   NA   NA
1336   1337   NA   NA   NA   NA
1338   1339   NA   NA   NA   NA
1340   1341   NA   NA   NA   NA
1342   1343   NA   NA   NA   NA
1344   1345   NA   NA   NA   NA
1346   1347   NA   NA   NA   NA
1348   1349   NA   NA   NA   NA
1350   1351   NA   NA   NA   NA
1352   1353   NA   NA   NA   NA
1354   1355   NA   NA   NA   NA
1356   1357   NA   NA   NA   NA
1358   1359   NA   NA   NA   NA
1360   1361   NA   NA   NA   NA
1362   1363   NA   NA   NA   NA
1364   1365   NA   NA   NA   NA
1366   1367   NA   NA   NA   NA
1368   1369   NA   NA   NA   NA
1370   1371   NA   NA   NA   NA
1372   1373   NA   NA   NA   NA
1374   1375   NA   NA   NA   NA
1376   1377   NA   NA   NA   NA
1378   1379   NA   NA   NA   NA
1380   1381   NA   NA   NA   NA
1382   1383   NA   NA   NA   NA
1384   1385   NA   NA   NA   NA
1386   1387   NA   NA   NA   NA
1388   1389   NA   NA   NA   NA
1390   1391   NA   NA   NA   NA
1392   1393   NA   NA   NA   NA
1394   1395   NA   NA   NA   NA
1396   1397   NA   NA   NA   NA
1398   1399   NA   NA   NA   NA
1400   1401   NA   NA   NA   NA
1402   1403   NA   NA   NA   NA
1404   1405   NA   NA   NA   NA
1406   1407   NA   NA   NA   NA
1408   1409   NA   NA   NA   NA
1410   1411   NA   NA   NA   NA
1412   1413   NA   NA   NA   NA
1414   1415   NA   NA   NA   NA
1416   1417   NA   NA   NA   NA
1418   1419   NA   NA   NA   NA
1420   1421   NA   NA   NA   NA
1422   1423   NA   NA   NA   NA
1424   1425   NA   NA   NA   NA
1426   1427   NA   NA   NA   NA
1428   1429   NA   NA   NA   NA
1430   1431   NA   NA   NA   NA
1432   1433   NA   NA   NA   NA
1434   1435   NA   NA   NA   NA
1436   1437   NA   NA   NA   NA
1438   1439   NA   NA   NA   NA
1440   1441   NA   NA   NA   NA
1442   1443   NA   NA   NA   NA
1444   1445   NA   NA   NA   NA
1446   1447   NA   NA   NA   NA
1448   1449   NA   NA   NA   NA
1450   1451   NA   NA   NA   NA
1452   1453   NA   NA   NA   NA
1454   1455   NA   NA   NA   NA
1456   1457   NA   NA   NA   NA
1458   1459   NA   NA   NA   NA
1460   1461   NA   NA   NA   NA
1462   1463   NA   NA   NA   NA
1464   1465   NA   NA   NA   NA
1466   1467   NA   NA   NA   NA
1468   1469   NA   NA   NA   NA
1470   1471   NA   NA   NA   NA
1472   1473   NA   NA   NA   NA
1474   1475   NA   NA   NA   NA
1476   1477   NA   NA   NA   NA
1478   1479   NA   NA   NA   NA
1480   1481   NA   NA   NA   NA
1482   1483   NA   NA   NA   NA
1484   1485   NA   NA   NA   NA
1486   1487   NA   NA   NA   NA
1488   1489   NA   NA   NA   NA
1490   1491   NA   NA   NA   NA
1492   1493   NA   NA   NA   NA
1494   1495   NA   NA   NA   NA
1496   1497   NA   NA   NA   NA
1498   1499   NA   NA   NA   NA
1500   1501   NA   NA   NA   NA
1502   1503   NA   NA   NA   NA
1504   1505   NA   NA   NA   NA
1506   1507   NA   NA   NA   NA
1508   1509   NA   NA   NA   NA
1510   1511   NA   NA   NA   NA
1512   1513   NA   NA   NA   NA
1514   1515   NA   NA   NA   NA
1516   1517   NA   NA   NA   NA
1518   1519   NA   NA   NA   NA
1520   1521   NA   NA   NA   NA
1522   1523   NA   NA   NA   NA
1524   1525   NA   NA   NA   NA
1526   1527   NA   NA   NA   NA
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| Models and submodels in the file (1453): lvc180axxxaaaaaaaain (Input), lvc180axxxbaaaaaaain (Input), lvc180axxxcaaaaaaain (Input), lvc180axxxdaaaaaaain (Input), lvc250axxxaaaaaaaain (Input), lvc250axxxbaaaaaaain (Input), lvc250axxxcaaaaaaain (Input), lvc250axxxdaaaaaaain (Input), lvc330axxxaaaaaaaain (Input), lvc330axxxbaaaaaaain (Input), lvc330axxxcaaaaaaain (Input), lvc330axxxdaaaaaaain (Input), lvc120axxxaaaaaaaain (Input), lvc120axxxbaaaaaaain (Input), lvc120axxxcaaaaaaain (Input), lvc120axxxdaaaaaaain (Input), lvc180f040aaaaaaaaou (Output), lvc180f080aaaaaaaaou (Output), lvc180f120aaaaaaaaou (Output), lvc180fr50aaaaaaaaou (Output), lvc180s040aaaaaaaaou (Output), lvc180s080aaaaaaaaou (Output), lvc180s120aaaaaaaaou (Output), lvc180sr50aaaaaaaaou (Output), lvc250f040aaaaaaaaou (Output), lvc250f080aaaaaaaaou (Output), lvc250f120aaaaaaaaou (Output), lvc250fr50aaaaaaaaou (Output), lvc250s040aaaaaaaaou (Output), lvc250s080aaaaaaaaou (Output), lvc250s120aaaaaaaaou (Output), lvc250sr50aaaaaaaaou (Output), lvc330f040aaaaaaaaou (Output), lvc330f080aaaaaaaaou (Output), lvc330f120aaaaaaaaou (Output), lvc330fr50aaaaaaaaou (Output), lvc330s040aaaaaaaaou (Output), lvc330s080aaaaaaaaou (Output), lvc330s120aaaaaaaaou (Output), lvc330sr50aaaaaaaaou (Output), lvc120f060aaaaaaaaou (Output), lvc120f080aaaaaaaaou (Output), lvc120s060aaaaaaaaou (Output), lvc120s080aaaaaaaaou (Output), lve250f120aaaaaaaaou (Output), lve250s120aaaaaaaaou (Output), sle180fr50aaaaaaaaou (Output), sle180sr50aaaaaaaaou (Output), lvc120axxxaaaaahaain (Input), lvc120axxxbaaaahaain (Input), lvc120axxxcaaaahaain (Input), lvc120axxxdaaaahaain (Input), lvc120axxxiaaaahaain (Input), lvc180axxxaaaaahaain (Input), lvc180axxxbaaaahaain (Input), lvc180axxxcaaaahaain (Input), lvc180axxxdaaaahaain (Input), lvc180axxxiaaaahaain (Input), lvc090axxxaaaaahaain (Input), lvc090axxxbaaaahaain (Input), lvc090axxxcaaaahaain (Input), lvc090axxxdaaaahaain (Input), lvc100axxxaaaaahaain (Input), lvc100axxxbaaaahaain (Input), lvc100axxxcaaaahaain (Input), lvc100axxxdaaaahaain (Input), lvc120f040aaaaahaaou (Output), lvc120f080aaaaahaaou (Output), lvc120f120aaaaahaaou (Output), lvc120s040aaaaahaaou (Output), lvc120s080aaaaahaaou (Output), lvc120s120aaaaahaaou (Output), lvc180f040aaaaahaaou (Output), lvc180f080aaaaahaaou (Output), lvc180f120aaaaahaaou (Output), lvc180fr50aaaaahaaou (Output), lvc180s040aaaaahaaou (Output), lvc180s080aaaaahaaou (Output), lvc180s120aaaaahaaou (Output), lvc180sr50aaaaahaaou (Output)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
